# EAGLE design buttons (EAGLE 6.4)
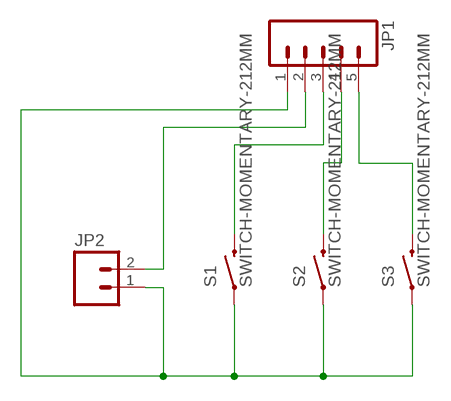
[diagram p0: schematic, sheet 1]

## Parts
JP1  M05LOCK_LONGPADS  [1X05_LOCK_LONGPADS]
JP2  M02PTH  [1X02]
S1  SWITCH-MOMENTARY-212MM  [TACTILE-PTH-12MM]
S2  SWITCH-MOMENTARY-212MM  [TACTILE-PTH-12MM]
S3  SWITCH-MOMENTARY-212MM  [TACTILE-PTH-12MM]

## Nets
N$1: JP1.5 S3.3
N$2: JP1.4 S2.3
N$3: JP1.3 S1.3
N$4: JP1.2 JP2.2
N$5: JP1.1 JP2.1 S1.1 S2.1 S3.1

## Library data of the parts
JP1 = SparkFun-Connectors:M05: Header 5 Standard 5-pin 0.1" header. Use with straight break away headers (SKU : PRT-00116), right angle break away headers (PRT-00553), swiss pins (PRT-00743), machine pins (PRT-00117), and female headers (PRT-00115). Molex polarized connector foot print use with SKU : PRT-08230 with associated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
JP2 = SparkFun-Connectors:M02: Header 2
S1-S3 = SparkFun-Electromechanical:SWITCH-MOMENTARY-2: Various NO switches- pushbuttons, reed, etc

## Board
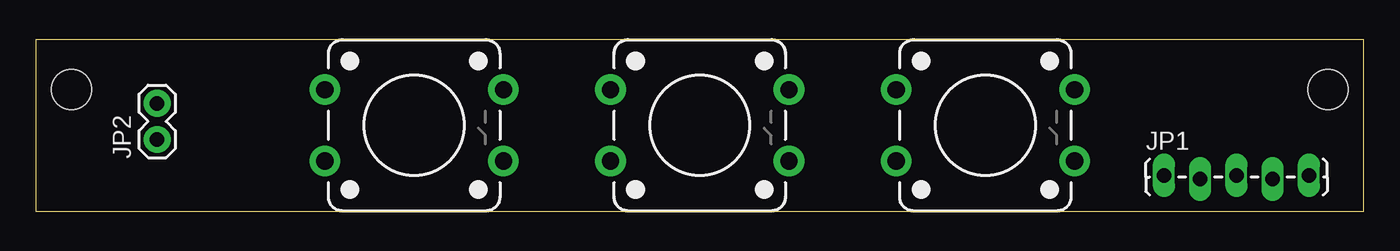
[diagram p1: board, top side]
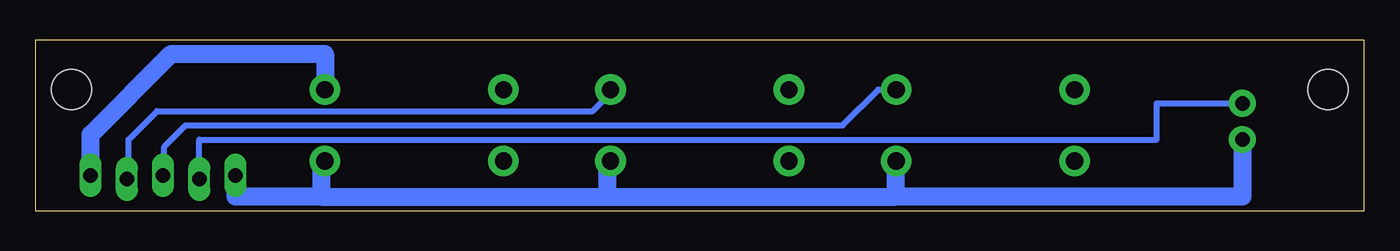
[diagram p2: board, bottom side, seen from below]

Size 93 x 12 mm. Coordinates in mm from the lower left corner, seen from the top.
Outline: 0,0 93,0 93,12 0,12 0,0
Copper layers (1*16): Top 0.035mm / dielectric 1.5mm / Bottom 0.035mm
Design rules "default": minimum track width 10mil, minimum drill 24mil, track to track 8mil, track to pad 8mil, pad to pad 8mil, via to via 8mil, smd to smd 8mil, copper to edge 40mil, drill to drill 8mil, minimum pad ring 10mil, minimum via ring 8mil, stop-mask expansion 4mil, vias tented up to drill 0mil, thermal gap 10mil
Holes 2.8 mm at 2.5,8.5 90.5,8.5

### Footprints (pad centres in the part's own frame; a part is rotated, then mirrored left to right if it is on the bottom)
1X05_LOCK_LONGPADS = drill 1.016 long: 1 0,0; 2 2.54,-0.254; 3 5.08,0; 4 7.62,-0.254; 5 10.16,0
1X02 = drill 1.016 pad 1.88: 1 0,0; 2 2.54,0
TACTILE-PTH-12MM = drill 1.2 pad 2.159: 1 6.25,-2.5; 2 -6.25,-2.5; 3 6.25,2.5; 4 -6.25,2.5

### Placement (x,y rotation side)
JP1  79,2.5 0 top
JP2  8.5,5 90 top
S1  26.5,6 0 top
S2  46.5,6 0 top
S3  66.5,6 0 top

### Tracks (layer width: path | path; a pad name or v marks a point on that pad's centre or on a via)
N$1
  Bottom 1.27: JP1.5 89.16,5.34 83.5,11 72.75,11 S3.3
N$2
  Bottom 0.406: JP1.4 86.5,2.25 86.5,5 84.5,7 54,7 52.75,8.25 S2.3
N$3
  Bottom 0.406: JP1.3 84,2.58 84,4.5 82.5,6 36.5,6 34,8.5 S1.3
N$4
  Bottom 0.406: JP1.2 81.54,5 14.5,5 14.5,7.54 JP2.2
N$5
  Bottom 1.27: JP2.1 8.5,1 32.75,1 | 32.75,1 S1.1 | S2.1 53,3.5 53,1 | 53,1 32.75,1 | 73,1 79,1 JP1.1 | S3.1 73,3.5 73,1 | 73,1 53,1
